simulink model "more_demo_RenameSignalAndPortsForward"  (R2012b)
settings: Solver=ode45  StartTime=0.0  StopTime=10.0  RelTol=1e-3

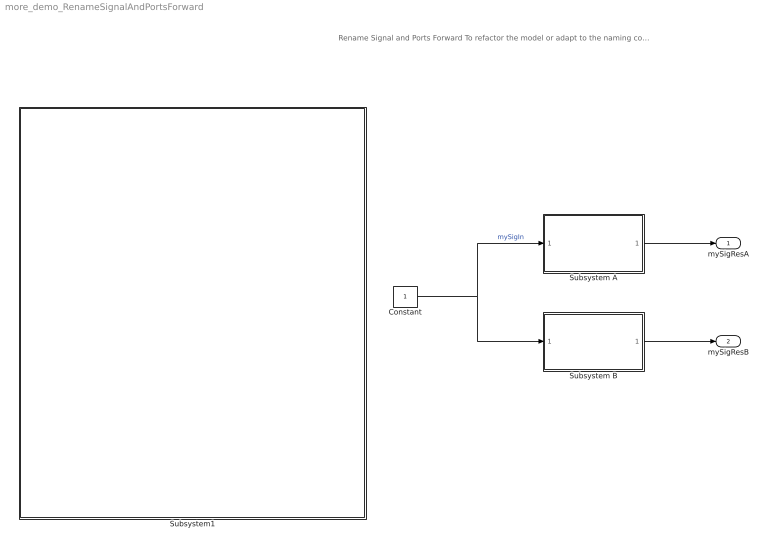
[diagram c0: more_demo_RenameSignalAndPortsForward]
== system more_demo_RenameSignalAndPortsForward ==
  note: Rename Signal and Ports Forward To refactor the model or adapt to the naming conventions, you may need to rename the signals and ports. The "Rename Signal and Ports" action makes this tedious task easier and faster.
  Constant : Constant
  Subsystem A : Subsystem
  Subsystem B : Subsystem
  Subsystem1 : Subsystem
  mySigResA : Outport
  mySigResB : Outport  Port=2
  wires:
  Constant/1 -> Subsystem A/1(mySigIn), Subsystem B/1(mySigIn)  "mySigIn"
  Subsystem B/1(mySigResB) -> mySigResB/1
  Subsystem A/1(mySigResA) -> mySigResA/1

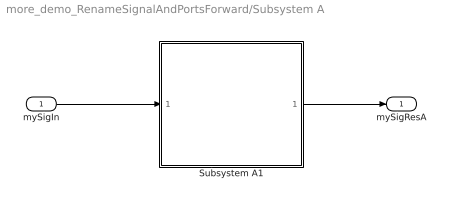
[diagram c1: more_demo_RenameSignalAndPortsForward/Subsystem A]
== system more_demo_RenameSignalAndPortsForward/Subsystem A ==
  mySigIn : Inport
  Subsystem A1 : Subsystem
  mySigResA : Outport
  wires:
  mySigIn/1 -> Subsystem A1/1(mySigIn)
  Subsystem A1/1(mySigResA) -> mySigResA/1

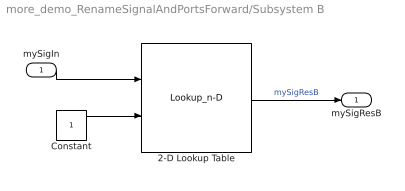
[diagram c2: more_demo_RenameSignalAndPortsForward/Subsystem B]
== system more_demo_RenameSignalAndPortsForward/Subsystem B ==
  mySigIn : Inport
  2-D Lookup Table : Lookup_n-D  BreakpointsForDimension1=[1:3]  BreakpointsForDimension2=[1:3]  RndMeth=Simplest
  Constant : Constant
  mySigResB : Outport
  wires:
  mySigIn/1 -> 2-D Lookup Table/1
  Constant/1 -> 2-D Lookup Table/2
  2-D Lookup Table/1 -> mySigResB/1  "mySigResB"

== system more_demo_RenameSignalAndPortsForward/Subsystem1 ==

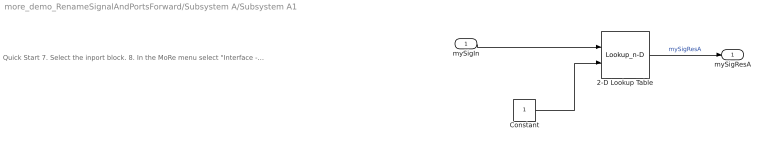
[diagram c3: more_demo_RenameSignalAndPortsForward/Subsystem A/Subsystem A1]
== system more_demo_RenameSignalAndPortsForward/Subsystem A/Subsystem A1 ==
  note: Quick Start 7. Select the inport block. 8. In the MoRe menu select "Interface -> Rename Signal and Ports Forward". 9. In the dialog set the option "Start At" to "Source of Signal". 10. Enter a name of your choice in the "New Name" field and select "Ok" in the dialog. 11. Check that the action has renamed the signal and all ports starting from the source block "Constant", which is located two levels higher. In particular, the action has also renamed ports located in "Subsystem B", which is in a different subtree than the selected element.
  mySigIn : Inport
  2-D Lookup Table : Lookup_n-D  BreakpointsForDimension1=[1:3]  BreakpointsForDimension2=[1:3]  RndMeth=Simplest
  Constant : Constant
  mySigResA : Outport
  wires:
  mySigIn/1 -> 2-D Lookup Table/1
  Constant/1 -> 2-D Lookup Table/2
  2-D Lookup Table/1 -> mySigResA/1  "mySigResA"
